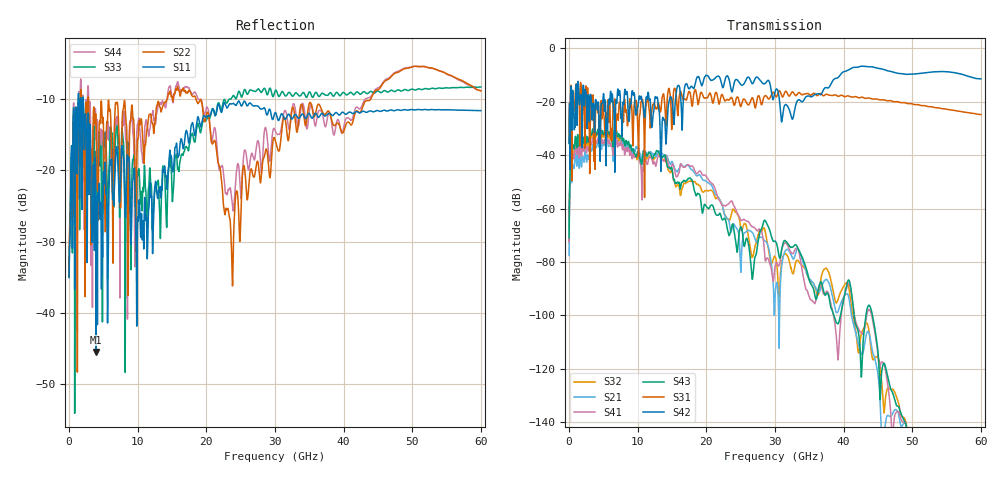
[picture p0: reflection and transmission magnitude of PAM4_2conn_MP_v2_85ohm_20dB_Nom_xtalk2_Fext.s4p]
! Info: Touchstone file created by Circ.  Input file=FAB50GbE_2conn_Midplane_Examax_Topo2_v2_85ohm_20dB_Nom.circ
# Hz S RI R 50
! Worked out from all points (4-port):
!   6000 points, 10 MHz to 60 GHz, reference 50 ohm
!   strongest paths, dB at 10 MHz, 15.01 GHz, 30.01 GHz, 45.01 GHz, 60 GHz:
!     S42: -35.6, -19.6, -16.3, -7.5, -11.4
!     S31: -35.4, -26.7, -17.5, -19.1, -24.8
!     S43: -71.0, -45.1, -72.2, -113.8, -160.8
!     S41: -72.2, -43.4, -81.7, -115.1, -169.6
!     S21: -77.6, -42.4, -93.3, -122.2, -168.3
!     S32: -73.0, -45.7, -77.9, -115.7, -154.1
!   lowest |S11| = -45.5 dB at 3.94 GHz (marker M1), VSWR 1.01, Z = 50.3 + j0.404 ohm
!   |S11| at or under -10 dB: start of sweep to 1.319 GHz; 1.733 GHz to 2.012 GHz (278.9 MHz wide, 14.9 % of centre); 2.075 GHz to end of sweep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
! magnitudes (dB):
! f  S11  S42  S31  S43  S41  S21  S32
! 10 MHz  -35.0  -35.6  -35.4  -71.0  -72.2  -77.6  -73.0
! 750 MHz  -14.9  -29.7  -21.4  -37.6  -41.0  -44.9  -39.2
! 3.94 GHz  -45.5  -19.5  -21.6  -32.3  -35.7  -37.2  -33.0
! 13.53 GHz  -22.8  -29.6  -18.9  -40.9  -41.7  -39.2  -41.2
! 26.71 GHz  -10.9  -13.2  -18.5  -86.5  -66.8  -69.0  -78.2
! 28.56 GHz  -11.4  -13.2  -17.7  -64.4  -79.0  -72.2  -68.2
! 60 GHz  -11.6  -11.4  -24.8  -160.8  -169.6  -168.3  -154.1
